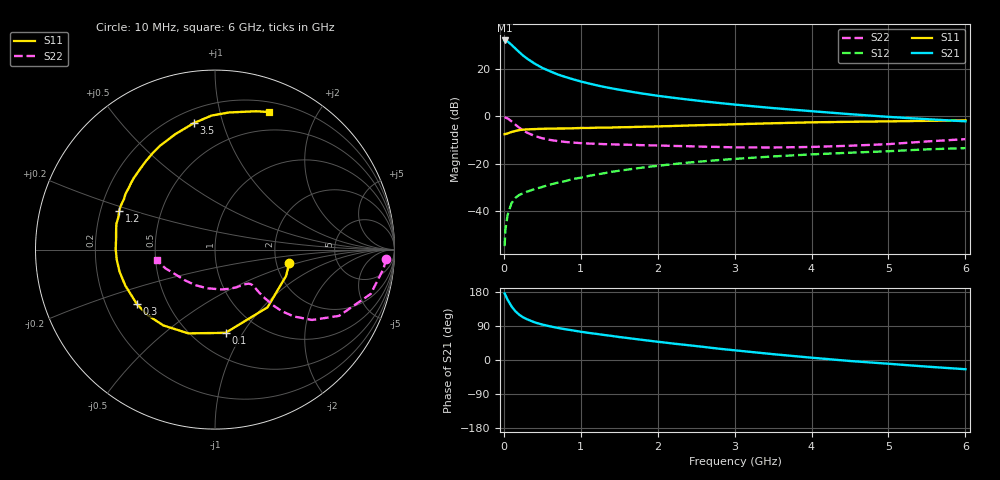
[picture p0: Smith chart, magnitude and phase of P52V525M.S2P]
! SIEMENS Small Signal Semiconductors
! BFP183
! Si NPN RF Bipolar Junction Transistor in SOT143
! VCE = 2.5 V  IC = 25 mA
! Common Emitter S-Parameters:  March  1996
# GHz  S  MA  R  50
!  f  S11  S21  S12  S22
! GHz  MAG  ANG  MAG  ANG  MAG  ANG  MAG  ANG
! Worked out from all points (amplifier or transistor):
!   36 points, 10 MHz to 6 GHz, reference 50 ohm
!   highest |S21| = 32.1 dB at 10 MHz (marker M1)
!   |S21| within 3 dB of that: start of sweep to 137 MHz
!   unconditionally stable (mu >= 1): 666.6 MHz to 5.564 GHz
!   at 250 MHz: K = 0.57, MSG = 29.1 dB, |S12| = -32.5 dB
!   at 1.4 GHz: K = 1.17, MAG = 15.2 dB, |S12| = -23.5 dB
!   at 6 GHz: K = 0.96, MSG = 5.7 dB, |S12| = -13.4 dB
!   S11 on the Smith chart (normalised r, x): 10 MHz: 2.36, -0.42; 100 MHz: 0.71, -0.84; 300 MHz: 0.33, -0.28; 1.2 GHz: 0.28, +0.18; 3.5 GHz: 0.28, +0.81; 6 GHz: 0.30, +1.43
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0.01  0.4208 -9.9  40.25 175.5  0.0018 87.5  0.9549 -3.1
0.02  0.4224 -20.2  40.14 171.5  0.004 81.8  0.9447 -6.5
0.05  0.4348 -47.7  38.22 158.7  0.0084 78.1  0.902 -15.9
0.1  0.4676 -82.8  32.49 141.6  0.0146 62.3  0.7837 -28.1
0.15  0.4899 -107.7  27.22 128.7  0.0189 55.8  0.6685 -35.9
0.2  0.5112 -124.3  22.8 119.6  0.0218 52.2  0.5763 -40.3
0.25  0.5241 -136.1  19.34 112.7  0.0236 50.3  0.5075 -42.6
0.3  0.5305 -145.1  16.75 107.6  0.0255 50.1  0.4536 -43.7
0.4  0.5384 -158.1  13.06 99.4  0.029 51.0  0.3854 -44.3
0.5  0.5461 -167.0  10.59 93.5  0.0322 51.0  0.3443 -44.2
0.6  0.5504 -174.4  8.99 88.8  0.036 52.2  0.3177 -43.8
0.7  0.5534 179.5  7.696 84.8  0.0396 54.4  0.3 -43.5
0.8  0.554 174.3  6.804 81.1  0.0428 54.5  0.2877 -43.5
1.1  0.5677 161.3  4.987 71.6  0.0549 55.7  0.2664 -45.4
1.2  0.5758 158.1  4.563 69.0  0.0587 55.4  0.2629 -46.5
1.7  0.5968 141.6  3.221 55.6  0.0784 53.8  0.2491 -54.1
2.2  0.6256 127.9  2.473 43.4  0.0977 50.4  0.237 -64.4
2.8  0.665 113.5  1.917 29.7  0.1192 44.9  0.2254 -80.0
3.5  0.7146 99.5  1.495 15.4  0.1421 38.7  0.2197 -101.4
4.5  0.7676 84.3  1.113 -2.6  0.1703 29.4  0.2393 -134.2
5.5  0.8043 73.4  0.872 -17.5  0.2007 21.3  0.2948 -159.1
6  0.8238 68.5  0.786 -24.3  0.2131 16.6  0.3298 -169.7
